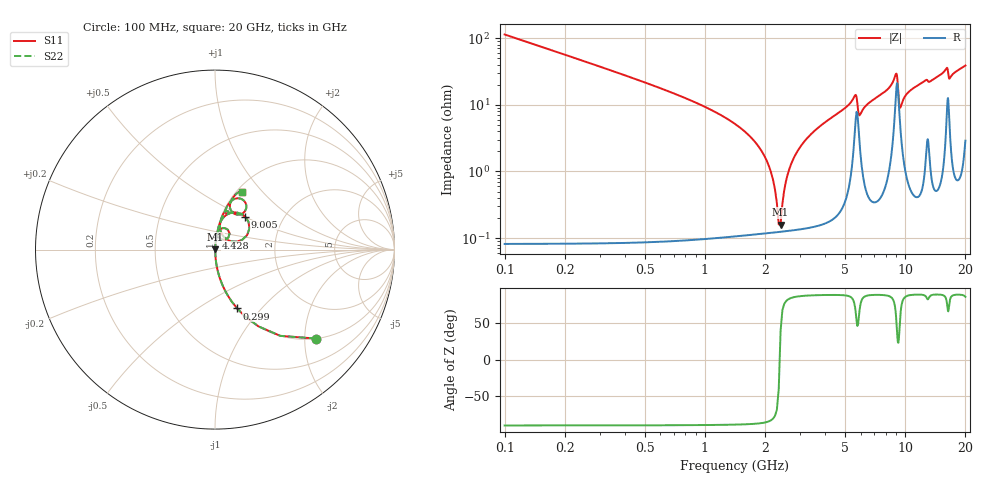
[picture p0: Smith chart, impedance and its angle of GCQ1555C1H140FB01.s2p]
!Murata Part Number: GCQ1555C1H140FB01
!These Parameters are Measured in Series Mode Connection
!Data Generated on Jan 08, 2026
!  o--ll--o
!Port1  Port2
!  o------o
!Operation Temp=25[degC], DC Bias Voltage=0[V]
!Freq. Start=100[MHz] Stop=20[GHz] 401[Steps]
# Hz S RI R 50
!Freq.(Hz) S11(Real) S11(Imag) S21(Real) S21(Imag) S12(Real) S12(Imag) S22(Real) S22(Imag)
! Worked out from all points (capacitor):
!   401 points, 100 MHz to 20 GHz, reference 50 ohm
!   read as one part in series: C = 14 pF near 199.5 MHz
!   lowest |Z| = 160 mohm at 2.389 GHz (marker M1)
!   series resonance near 2.364 GHz, so ESL is about 320 pH
!   S11 on the Smith chart (normalised r, x): 100 MHz: 1.00, -2.27; 299 MHz: 1.00, -0.75; 4.428 GHz: 1.00, +0.14; 9.005 GHz: 1.29, +0.51; 20 GHz: 1.06, +0.77
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1e8  0.5628 -0.4957  0.4372 0.4957  0.4372 0.4957  0.5628 -0.4957
2.99e8  0.1233 -0.3277  0.8767 0.3277  0.8767 0.3277  0.1233 -0.3277
7.965e8  0.0166 -0.1243  0.9834 0.1243  0.9834 0.1243  0.0166 -0.1243
1.84125e9  0.00174 -0.0243  0.9983 0.0243  0.9983 0.0243  0.00174 -0.0243
2.09e9  0.00133 -0.0119  0.9987 0.0119  0.9987 0.0119  0.00133 -0.0119
2.289e9  0.00124 -0.00311  0.9988 0.00311  0.9988 0.00311  0.00124 -0.00311
2.3885e9  0.00125 0.001  0.9988 -0.001  0.9988 -0.001  0.00125 0.001
2.5875e9  0.00136 0.00877  0.9986 -0.00877  0.9986 -0.00877  0.00136 0.00877
2.73675e9  0.00151 0.0143  0.9985 -0.0143  0.9985 -0.0143  0.00151 0.0143
3.43325e9  0.00286 0.0375  0.9971 -0.0375  0.9971 -0.0375  0.00286 0.0375
4.42825e9  0.00663 0.0679  0.9934 -0.0679  0.9934 -0.0679  0.00663 0.0679
5.5725e9  0.0437 0.1198  0.9563 -0.1198  0.9563 -0.1198  0.0437 0.1198
5.92075e9  0.0302 0.0604  0.9698 -0.0604  0.9698 -0.0604  0.0302 0.0604
6.7665e9  0.0161 0.1109  0.9839 -0.1109  0.9839 -0.1109  0.0161 0.1109
8.458e9  0.048 0.1798  0.952 -0.1798  0.952 -0.1798  0.048 0.1798
9.00525e9  0.168 0.1834  0.832 -0.1834  0.832 -0.1834  0.168 0.1834
9.40325e9  0.0612 0.06  0.9388 -0.06  0.9388 -0.06  0.0612 0.06
1.005e10  0.0276 0.1323  0.9724 -0.1323  0.9724 -0.1323  0.0276 0.1323
1.338325e10  0.0579 0.2107  0.9421 -0.2107  0.9421 -0.2107  0.0579 0.2107
1.606975e10  0.1431 0.2835  0.8569 -0.2835  0.8569 -0.2835  0.1431 0.2835
1.67165e10  0.0906 0.2154  0.9094 -0.2154  0.9094 -0.2154  0.0906 0.2154
2e10  0.1483 0.3199  0.8517 -0.3199  0.8517 -0.3199  0.1483 0.3199
